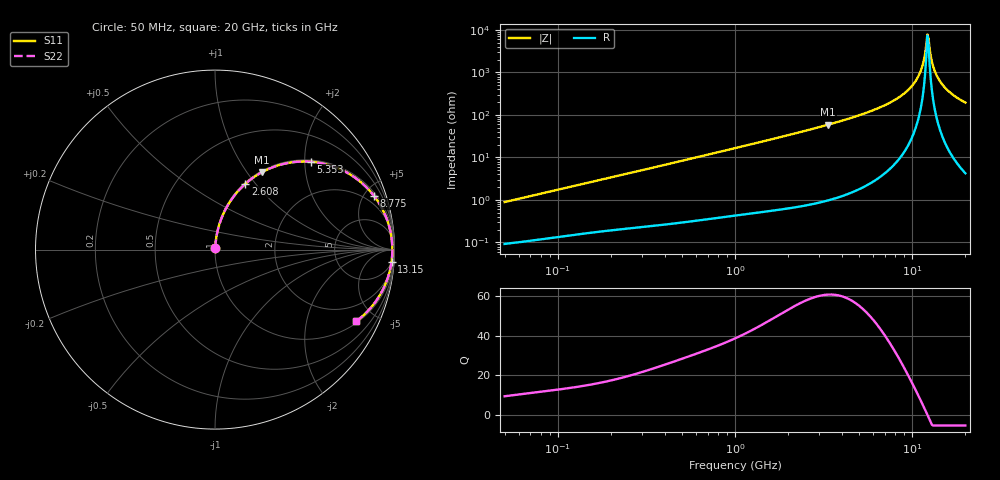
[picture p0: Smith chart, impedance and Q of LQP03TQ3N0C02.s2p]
!Murata Part Number: LQP03TQ3N0C02
!These Parameters are Measured in Series Mode Connection
!  o--[Z]--o
!Port1  Port2
!  o-------o
!Freq. Start=50[MHz] Stop=20[GHz], 401[Steps]
# Hz S RI R 50
!Freq.(Hz) S11(Real) S11(Imag) S21(Real) S21(Imag) S12(Real) S12(Imag) S22(Real) S22(Imag)
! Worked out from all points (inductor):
!   401 points, 50 MHz to 20 GHz, reference 50 ohm
!   read as one part in series: L = 2.79 nH near 51.52 MHz
!   highest Q = 60.5 at 3.364 GHz (marker M1), where L = 2.79 nH
!   self-resonance near 12.2 GHz
!   S11 on the Smith chart (normalised r, x): 50 MHz: 1.00, +0.02; 2.608 GHz: 1.02, +0.89; 5.353 GHz: 1.04, +2.14; 8.775 GHz: 1.23, +5.83; 13.15 GHz: 6, -27; 20 GHz: 1.08, -3.89
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5e7  0.000998 0.00883  0.999 -0.00883  0.999 -0.00883  0.000998 0.00883
1.364002e8  0.00213 0.0232  0.9979 -0.0232  0.9979 -0.0232  0.00213 0.0232
3.721004e8  0.00632 0.0614  0.9937 -0.0614  0.9937 -0.0614  0.00632 0.0614
1e9  0.0304 0.1592  0.9696 -0.1592  0.9696 -0.1592  0.0304 0.1592
2.608132e9  0.1688 0.3661  0.8312 -0.3661  0.8312 -0.3661  0.1688 0.3661
2.728004e9  0.1827 0.378  0.8173 -0.378  0.8173 -0.378  0.1827 0.378
3.364474e9  0.262 0.4316  0.738 -0.4316  0.738 -0.4316  0.262 0.4316
5.352748e9  0.5343 0.4894  0.4657 -0.4894  0.4657 -0.4894  0.5343 0.4894
7.442007e9  0.7787 0.4017  0.2213 -0.4017  0.2213 -0.4017  0.7787 0.4017
8.774992e9  0.8857 0.2994  0.1143 -0.2994  0.1143 -0.2994  0.8857 0.2994
9.892087e9  0.944 0.2025  0.056 -0.2025  0.056 -0.2025  0.944 0.2025
1.082228e10  0.9728 0.1206  0.0272 -0.1206  0.0272 -0.1206  0.9728 0.1206
1.131968e10  0.9818 0.0776  0.0182 -0.0776  0.0182 -0.0776  0.9818 0.0776
1.201863e10  0.9877 0.0191  0.0123 -0.0191  0.0123 -0.0191  0.9877 0.0191
1.220001e10  0.9881 0.00436  0.0119 -0.00436  0.0119 -0.00436  0.9881 0.00436
1.238412e10  0.9881 -0.0104  0.0119 0.0104  0.0119 0.0104  0.9881 -0.0104
1.257102e10  0.9876 -0.0251  0.0124 0.0251  0.0124 0.0251  0.9876 -0.0251
1.314879e10  0.9835 -0.069  0.0165 0.069  0.0165 0.069  0.9835 -0.069
1.396067e10  0.972 -0.1265  0.028 0.1265  0.028 0.1265  0.972 -0.1265
1.527346e10  0.9426 -0.2083  0.0574 0.2083  0.0574 0.2083  0.9426 -0.2083
1.721783e10  0.8835 -0.305  0.1165 0.305  0.1165 0.305  0.8835 -0.305
2e10  0.7864 -0.3992  0.2136 0.3992  0.2136 0.3992  0.7864 -0.3992
